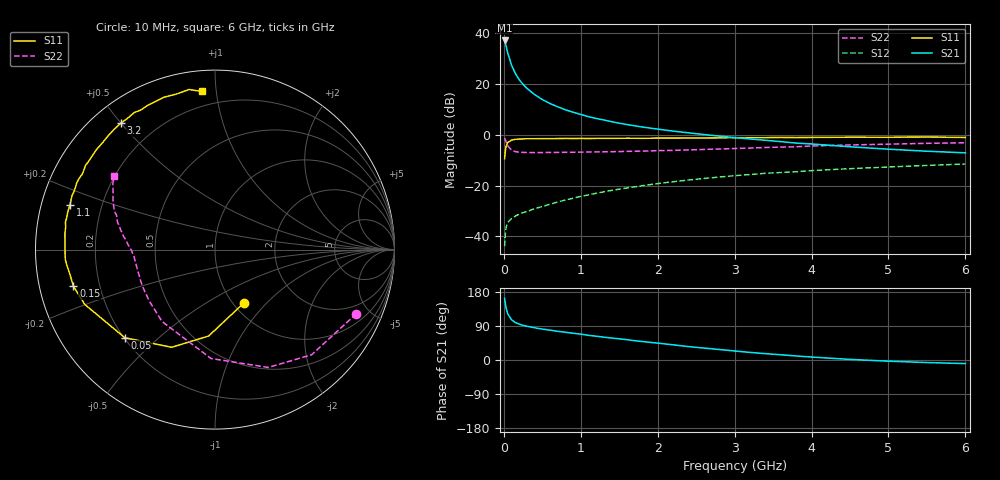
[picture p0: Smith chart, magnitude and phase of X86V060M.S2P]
! SIEMENS Small Signal Semiconductors
! BFP136W
! Si NPN RF Bipolar Junction Transistor in SOT343
! VCE = 6 V  IC = 60 mA
! Common Emitter S-Parameters:  September  1994
# GHz  S  MA  R  50
!  f  S11  S21  S12  S22
! GHz  MAG  ANG  MAG  ANG  MAG  ANG  MAG  ANG
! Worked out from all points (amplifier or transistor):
!   40 points, 10 MHz to 6 GHz, reference 50 ohm
!   highest |S21| = 37.1 dB at 10 MHz (marker M1)
!   |S21| within 3 dB of that: start of sweep to 35.84 MHz
!   unconditionally stable (mu >= 1): 691.5 MHz to 2.944 GHz
!   at 200 MHz: K = 0.57, MSG = 26.5 dB, |S12| = -31.2 dB
!   at 1.5 GHz: K = 1.11, MAG = 11.0 dB, |S12| = -21.4 dB
!   at 6 GHz: K = 0.96, MSG = 2.2 dB, |S12| = -11.5 dB
!   S11 on the Smith chart (normalised r, x): 10 MHz: 1.12, -0.75; 50 MHz: 0.20, -0.39; 150 MHz: 0.10, -0.13; 1.1 GHz: 0.09, +0.15; 3.2 GHz: 0.08, +0.50; 6 GHz: 0.11, +0.91
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0.01  0.3377 -61.5  72 162.8  0.0064 72.4  0.8648 -24.4
0.02  0.4828 -94.2  63.72 148.0  0.0113 61.3  0.7957 -47.4
0.03  0.5953 -113.9  55.63 136.8  0.0149 53.3  0.7204 -65.7
0.05  0.7024 -135.6  41.23 122.1  0.0187 40.4  0.6071 -92.1
0.1  0.7868 -157.1  23.47 106.1  0.0224 34.6  0.4976 -126.4
0.15  0.8149 -165.5  16.1 98.9  0.0251 34.4  0.4649 -142.0
0.2  0.8199 -170.3  12.14 94.6  0.0274 35.7  0.4541 -150.8
0.25  0.8301 -174.0  9.813 91.4  0.0293 37.9  0.4501 -156.5
0.3  0.836 -176.3  8.214 89.1  0.0308 39.4  0.4468 -160.2
0.4  0.8357 179.5  6.191 85.0  0.0351 42.9  0.4465 -165.3
0.5  0.8374 176.4  4.944 81.6  0.0387 46.1  0.447 -168.7
0.6  0.8408 174.1  4.121 78.8  0.0429 48.3  0.4483 -170.8
0.7  0.8416 171.4  3.556 75.7  0.0473 50.4  0.4499 -172.3
0.8  0.8473 169.5  3.11 73.2  0.052 52.4  0.4513 -173.8
0.9  0.845 167.6  2.779 70.6  0.0562 53.2  0.4525 -175.1
1.1  0.8453 163.0  2.274 65.1  0.0656 54.9  0.4576 -176.8
1.5  0.8509 156.2  1.69 55.9  0.0849 55.9  0.4668 -179.8
2.2  0.8593 143.7  1.181 40.1  0.1187 52.9  0.4928 175.1
3.2  0.878 126.7  0.826 20.1  0.1649 45.3  0.5474 166.4
4.5  0.8953 108.6  0.58 1.6  0.2151 34.1  0.63 154.4
5.5  0.9035 99.2  0.474 -6.7  0.249 26.2  0.6784 147.0
6  0.8846 94.8  0.441 -9.5  0.2658 21.9  0.6963 143.9
